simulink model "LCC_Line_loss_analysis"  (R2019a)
settings: Solver=VariableStepAuto  StartTime=0.0  StopTime=10.0  RelTol=1e-3
undefined symbols (not defined in the file or in its folder): D1, Delta
libraries: powerlib x40, powerlib_meascontrol x15

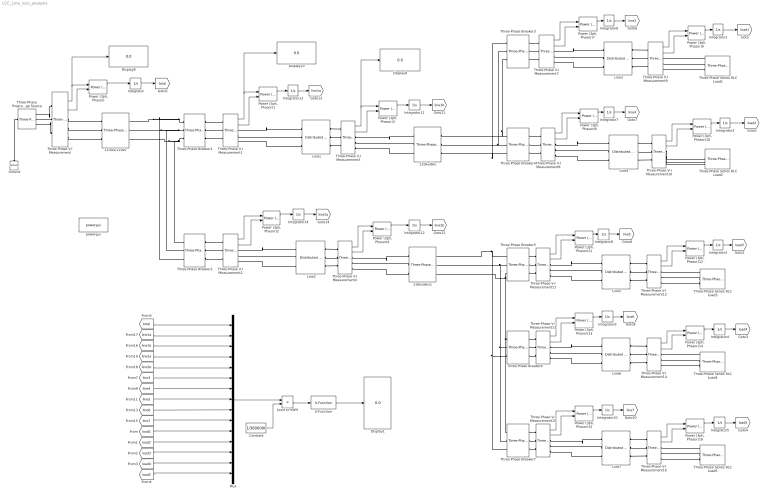
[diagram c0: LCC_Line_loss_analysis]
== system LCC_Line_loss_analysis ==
  " Line1" : powerlib/Elements/Distributed Parameters Line  Phases=3  Frequency=50  Resistance=[0.01273 0.3864]  Inductance="[0.9337e-3  4.1264e-3]"  Capacitance=[12.74e-9 7.751e-9]  Length=50  x1=[2.42627004663306e-09 109999.988635865 109999.988635865;314.159265358979 314.159265358979 314.159265358979;1.80703091597691 0.469420595754554 -1.10137573104034]  x2=[2.86623095915016e-09 110162.552221419 110162.552221419;314.159265358979 314.159265358979 314.159265358979;1.78484613356119 0.469205113607915 -1.10159121318698]  x3=[7.23800122018368e-12 405.078766721455 405.078766721459;314.159265358979 314.159265358979 314.159265358979;0.785734525687869 0.414782441285651 -1.15601388550923]  x4=[7.02816694582336e-12 407.341080813924 407.341080813919;314.159265358979 314.159265358979 314.159265358979;2.98486211281806 0.469482730989694 -1.10131359580521]  x5=0.000282770783497871  V1=[2.426e-09 1.1e+05 1.1e+05;314.2 314.2 314.2;1.807 0.4694 -1.101]  V2=[2.866e-09 1.102e+05 1.102e+05;314.2 314.2 314.2;1.785 0.4692 -1.102]  I1=[7.238e-12 405.1 405.1;314.2 314.2 314.2;0.7857 0.4148 -1.156]  I2=[7.028e-12 407.3 407.3;314.2 314.2 314.2;2.985 0.4695 -1.101]  nHarmo=1  Measurements=None
  " Line2" : powerlib/Elements/Distributed Parameters Line  Phases=3  Frequency=50  Resistance=[0.01273 0.3864]  Inductance="[0.9337e-3  4.1264e-3]"  Capacitance=[12.74e-9 7.751e-9]  Length=50  x1=[2.41365569055271e-09 109999.984096595 109999.984096595;314.159265358979 314.159265358979 314.159265358979;1.810384742463 1.51661814213263 3.08741446892753]  x2=[2.30050693096151e-09 110163.037727826 110163.037727826;314.159265358979 314.159265358979 314.159265358979;1.79045646876788 1.51634195109301 3.08713827788791]  x3=[2.00567277565264e-12 404.628931687138 404.628931687133;314.159265358979 314.159265358979 314.159265358979;2.27601187025823 1.46178814856789 3.03258447536278]  x4=[4.11611761403107e-12 407.795592688783 407.795592688789;314.159265358979 314.159265358979 314.159265358979;1.4069351072644 1.51674944032911 3.08754576712401]  x5=0.000282770783497871  V1=[2.414e-09 1.1e+05 1.1e+05;314.2 314.2 314.2;1.81 1.517 3.087]  V2=[2.301e-09 1.102e+05 1.102e+05;314.2 314.2 314.2;1.79 1.516 3.087]  I1=[2.006e-12 404.6 404.6;314.2 314.2 314.2;2.276 1.462 3.033]  I2=[4.116e-12 407.8 407.8;314.2 314.2 314.2;1.407 1.517 3.088]  nHarmo=1  Measurements=None
  " Line3" : powerlib/Elements/Distributed Parameters Line  Phases=3  Frequency=50  Resistance=[0.01273 0.3864]  Inductance="[0.9337e-3  4.1264e-3]"  Capacitance=[12.74e-9 7.751e-9]  Length=50  x1=[7.59305529381592e-11 6008.18273156121 6008.18273156127;314.159265358979 314.159265358979 314.159265358979;1.15263509813838 0.991548021886359 2.56234434868125]  x2=[6.89253585630512e-11 6010.19477333752 6010.19477333757;314.159265358979 314.159265358979 314.159265358979;1.12473499523216 0.971117638857499 2.54191396565239]  x3=[1.12891283616764e-13 13.8436307559632 13.8436307559631;314.159265358979 314.159265358979 314.159265358979;2.02903845670185 0.918213317671723 2.48900964446667]  x4=[1.94803250183711e-13 30.4994291398562 30.4994291398567;314.159265358979 314.159265358979 314.159265358979;0.741119579924984 0.970570895126736 2.54136722192161]  x5=0.000282770783497871  V1=[7.593e-11 6008 6008;314.2 314.2 314.2;1.153 0.9915 2.562]  V2=[6.893e-11 6010 6010;314.2 314.2 314.2;1.125 0.9711 2.542]  I1=[1.129e-13 13.84 13.84;314.2 314.2 314.2;2.029 0.9182 2.489]  I2=[1.948e-13 30.5 30.5;314.2 314.2 314.2;0.7411 0.9706 2.541]  nHarmo=1  Measurements=None
  " Line4" : powerlib/Elements/Distributed Parameters Line  Phases=3  Frequency=50  Resistance=[0.01273 0.3864]  Inductance="[0.9337e-3  4.1264e-3]"  Capacitance=[12.74e-9 7.751e-9]  Length=100  x1=[7.70769930533368e-11 6008.14875836645 6008.14875836645;314.159265358979 314.159265358979 314.159265358979;0.92815933412839 -0.109826923976571 -1.68062325077146]  x2=[5.61940897329232e-11 6019.23621249713 6019.23621249713;314.159265358979 314.159265358979 314.159265358979;0.4847481944804 -0.167146792126099 -1.73794311892099]  x3=[1.60493033480814e-13 10.5340155159656 10.5340155159655;314.159265358979 314.159265358979 314.159265358979;-3.0013468861881 -0.276666920445539 -1.84746324724043]  x4=[3.57813419959134e-13 33.8325750993465 33.8325750993465;314.159265358979 314.159265358979 314.159265358979;0.332480731404384 -0.166653751439935 -1.73745007823482]  x5=0.000565541566995743  V1=[7.708e-11 6008 6008;314.2 314.2 314.2;0.9282 -0.1098 -1.681]  V2=[5.619e-11 6019 6019;314.2 314.2 314.2;0.4847 -0.1671 -1.738]  I1=[1.605e-13 10.53 10.53;314.2 314.2 314.2;-3.001 -0.2767 -1.847]  I2=[3.578e-13 33.83 33.83;314.2 314.2 314.2;0.3325 -0.1667 -1.737]  nHarmo=1  Measurements=None
  " Line5" : powerlib/Elements/Distributed Parameters Line  Phases=3  Frequency=50  Resistance=[0.01273 0.3864]  Inductance="[0.9337e-3  4.1264e-3]"  Capacitance=[12.74e-9 7.751e-9]  Length=70  x1=[2.06803460954251e-11 6008.01639533854 6008.01639533867;314.159265358979 314.159265358979 314.159265358979;-1.55026791798683 2.01650369223936 -2.69588528814532]  x2=[3.29966131788237e-11 6022.29777272544 6022.29777272558;314.159265358979 314.159265358979 314.159265358979;-2.21431152729356 2.00495247781881 -2.70743650256587]  x3=[2.18092693874683e-13 18.8614244081539 18.8614244081542;314.159265358979 314.159265358979 314.159265358979;2.19365442019187 1.92830769506266 -2.78408128532201]  x4=[2.40433029961128e-13 25.5309379087104 25.5309379087111;314.159265358979 314.159265358979 314.159265358979;-1.27694108346781 2.00560662914093 -2.70678235124375]  x5=0.00039587909689702  V1=[2.068e-11 6008 6008;314.2 314.2 314.2;-1.55 2.017 -2.696]  V2=[3.3e-11 6022 6022;314.2 314.2 314.2;-2.214 2.005 -2.707]  I1=[2.181e-13 18.86 18.86;314.2 314.2 314.2;2.194 1.928 -2.784]  I2=[2.404e-13 25.53 25.53;314.2 314.2 314.2;-1.277 2.006 -2.707]  nHarmo=1  Measurements=None
  " Line6" : powerlib/Elements/Distributed Parameters Line  Phases=3  Frequency=50  Resistance=[0.01273 0.3864]  Inductance="[0.9337e-3  4.1264e-3]"  Capacitance=[12.74e-9 7.751e-9]  Length=75  x1=[1.90824246118878e-11 6007.96613140158 6007.96613140145;314.159265358979 314.159265358979 314.159265358979;-1.26596522315896 0.963888688570127 -0.606907638224758]  x2=[2.76583978250132e-11 6017.39726878102 6017.3972687809;314.159265358979 314.159265358979 314.159265358979;-2.1640200741846 0.933168217076156 -0.637628109718729]  x3=[1.91761145536608e-13 13.8552900858033 13.8552900858031;314.159265358979 314.159265358979 314.159265358979;2.06333552307775 0.850861543484025 -0.719934783310865]  x4=[2.45843562433831e-13 30.5115242564101 30.5115242564094;314.159265358979 314.159265358979 314.159265358979;-1.11015247428008 0.933715077486628 -0.637081249308253]  x5=0.000424156175246807  V1=[1.908e-11 6008 6008;314.2 314.2 314.2;-1.266 0.9639 -0.6069]  V2=[2.766e-11 6017 6017;314.2 314.2 314.2;-2.164 0.9332 -0.6376]  I1=[1.918e-13 13.86 13.86;314.2 314.2 314.2;2.063 0.8509 -0.7199]  I2=[2.458e-13 30.51 30.51;314.2 314.2 314.2;-1.11 0.9337 -0.6371]  nHarmo=1  Measurements=None
  " Line7" : powerlib/Elements/Distributed Parameters Line  Phases=3  Frequency=50  Resistance=[0.01273 0.3864]  Inductance="[0.9337e-3  4.1264e-3]"  Capacitance=[12.74e-9 7.751e-9]  Length=50  x1=[1.81374523428606e-11 6007.88313297421 6007.88313297408;314.159265358979 314.159265358979 314.159265358979;-1.10950345529888 0.990978480375292 -0.579817846419593]  x2=[2.19506880714965e-11 6001.34524535515 6001.34524535502;314.159265358979 314.159265358979 314.159265358979;-1.88953581653548 0.950225697994974 -0.620570628799912]  x3=[1.88636400080801e-13 5.51740302808399 5.51740302808387;314.159265358979 314.159265358979 314.159265358979;2.24025021280838 0.893262455463956 -0.677533871330898]  x4=[2.46025626104762e-13 38.77992905964 38.7799290596392;314.159265358979 314.159265358979 314.159265358979;-1.06174768352794 0.950655064902487 -0.620141261892399]  x5=0.000282770783497871  V1=[1.814e-11 6008 6008;314.2 314.2 314.2;-1.11 0.991 -0.5798]  V2=[2.195e-11 6001 6001;314.2 314.2 314.2;-1.89 0.9502 -0.6206]  I1=[1.886e-13 5.517 5.517;314.2 314.2 314.2;2.24 0.8933 -0.6775]  I2=[2.46e-13 38.78 38.78;314.2 314.2 314.2;-1.062 0.9507 -0.6201]  nHarmo=1  Measurements=None
  110kv/6kv : powerlib/Elements/Three-Phase Transformer (Two Windings)  Winding1Connection=Yg  Winding2Connection=Delta (D1)  CoreType=Three single-phase transformers  SetSaturation=off  Hysteresis=off  DataFile='hysteresis'  SetInitialFlux=off  Measurements=None  UNITS=pu  NominalPower=[ 2e6 , 50 ]  Winding1=[ 110e3 , 0.002 , 0.01]  Winding2=[ 6000 , 0.002 , 0.01]  Rm=500  Lm=500  L0=0.5  Saturation=[ 0,0 ; 0.0024,1.2 ; 1.0,1.52 ]  InitialFluxes=[ 0.8 , -0.8 , 0.7 ]  BreakLoop=off  DiscreteSolver=Trapezoidal iterative  DataType=off  TransfoNumber=1
  110kv/6kv1 : powerlib/Elements/Three-Phase Transformer (Two Windings)  Winding1Connection=Yg  Winding2Connection=Delta (D1)  CoreType=Three single-phase transformers  SetSaturation=off  Hysteresis=off  DataFile='hysteresis'  SetInitialFlux=off  Measurements=None  UNITS=pu  NominalPower=[ 2e6 , 50 ]  Winding1=[ 110e3 , 0.002 , 0.01]  Winding2=[ 6000 , 0.002 , 0.01]  Rm=500  Lm=500  L0=0.5  Saturation=[ 0,0 ; 0.0024,1.2 ; 1.0,1.52 ]  InitialFluxes=[ 0.8 , -0.8 , 0.7 ]  BreakLoop=off  DiscreteSolver=Trapezoidal iterative  DataType=off  TransfoNumber=1
  13.6kv/110kv : powerlib/Elements/Three-Phase Transformer (Two Windings)  Winding1Connection=Y  Winding2Connection=Yg  CoreType=Three single-phase transformers  SetSaturation=off  Hysteresis=off  DataFile='hysteresis'  SetInitialFlux=off  Measurements=None  UNITS=pu  NominalPower=[ 4e6 , 50 ]  Winding1=[ 13600 , 0 , 0]  Winding2=[ 110e3 , 0 , 0]  Rm=inf  Lm=inf  L0=0.5  Saturation=[ 0,0 ; 0.0024,1.2 ; 1.0,1.52 ]  InitialFluxes=[ 0.8 , -0.8 , 0.7 ]  BreakLoop=off  DiscreteSolver=Trapezoidal iterative  DataType=off  TransfoNumber=1
  Constant : Constant  Value=1/3600000
  Display{1,8..10} (4 alike) : Display
  Ground : powerlib/Elements/Ground  LConnTagsString=a
  Integrator{,1..14} (15 alike) : Integrator
  Joule to KWH : Product
  Mux : Mux  Inputs=15
  Power (3ph, Phasor){,1..4,7..16} (15 alike) : powerlib_meascontrol/Measurements/Power (3ph, Phasor)
  S-Function : S-Function  FunctionName=modbusCom2  SFunctionDeploymentMode=off  EnableBusSupport=off
  Three-Phase Programmable Voltage Source : powerlib/Electrical Sources/Three-Phase Programmable Voltage Source  PositiveSequence="[13.6e3  0 50]"  VariationEntity=None  VariationType=Step  VariationTypeAlt=Step  VariationStep=-0.6  VariationRate=10  VariationMagnitude=0.3  VariationFrequency=2  VariationTiming=[20 30]  VariationPhaseA=off  Amplitudes=[1 0.8 1.2 1.0]  TimeValues=[0 0.1 0.15 0.2]  HarmonicGeneration=off  HarmonicA=[3 0.2 -25 0]  HarmonicB=[2 0.15 35 2]  Timing="[0.05  3]"  BusType=swing  Pref=0  Qref=0  Qmin=-inf  Qmax=inf
  Three-Phase Series RLC Load1 : powerlib/Elements/Three-Phase Series RLC Load  LConnTagsString=A|B|C  Configuration=Y (grounded)  NominalVoltage=6000  Vabc=[1e3 1e3 1e3]  Vabcp=[1e3 1e3 1e3]  NominalFrequency=50  UnbalancedPower=off  ActivePower=50000  InductivePower=100  CapacitivePower=0  Pabc=[10e3 9e3 11e3]  QLabc=[100 90 110]  QCabc=[100 90 110]  Pabcp=[10e3 9e3 11e3]  QLabcp=[100 90 110]  QCabcp=[100 90 110]  Measurements=None  LoadType=constant Z
  Three-Phase Series RLC Load2 : powerlib/Elements/Three-Phase Series RLC Load  LConnTagsString=A|B|C  Configuration=Y (grounded)  NominalVoltage=6000  Vabc=[1e3 1e3 1e3]  Vabcp=[1e3 1e3 1e3]  NominalFrequency=50  UnbalancedPower=off  ActivePower=70000  InductivePower=0  CapacitivePower=100  Pabc=[10e3 9e3 11e3]  QLabc=[100 90 110]  QCabc=[100 90 110]  Pabcp=[10e3 9e3 11e3]  QLabcp=[100 90 110]  QCabcp=[100 90 110]  Measurements=None  LoadType=constant PQ
  Three-Phase Series RLC Load3 : powerlib/Elements/Three-Phase Series RLC Load  LConnTagsString=A|B|C  Configuration=Y (grounded)  NominalVoltage=6000  Vabc=[1e3 1e3 1e3]  Vabcp=[1e3 1e3 1e3]  NominalFrequency=50  UnbalancedPower=off  ActivePower=20000  InductivePower=0  CapacitivePower=100  Pabc=[10e3 9e3 11e3]  QLabc=[100 90 110]  QCabc=[100 90 110]  Pabcp=[10e3 9e3 11e3]  QLabcp=[100 90 110]  QCabcp=[100 90 110]  Measurements=None  LoadType=constant Z
  Three-Phase Series RLC Load4 : powerlib/Elements/Three-Phase Series RLC Load  LConnTagsString=A|B|C  Configuration=Y (grounded)  NominalVoltage=6000  Vabc=[1e3 1e3 1e3]  Vabcp=[1e3 1e3 1e3]  NominalFrequency=50  UnbalancedPower=off  ActivePower=50000  InductivePower=0  CapacitivePower=100  Pabc=[10e3 9e3 11e3]  QLabc=[100 90 110]  QCabc=[100 90 110]  Pabcp=[10e3 9e3 11e3]  QLabcp=[100 90 110]  QCabcp=[100 90 110]  Measurements=None  LoadType=constant Z
  Three-Phase Series RLC Load5 : powerlib/Elements/Three-Phase Series RLC Load  LConnTagsString=A|B|C  Configuration=Y (grounded)  NominalVoltage=6000  Vabc=[1e3 1e3 1e3]  Vabcp=[1e3 1e3 1e3]  NominalFrequency=50  UnbalancedPower=off  ActivePower=100000  InductivePower=0  CapacitivePower=100  Pabc=[10e3 9e3 11e3]  QLabc=[100 90 110]  QCabc=[100 90 110]  Pabcp=[10e3 9e3 11e3]  QLabcp=[100 90 110]  QCabcp=[100 90 110]  Measurements=None  LoadType=constant Z
  Three-Phase V-I Measurement{,1..4,7..16} (15 alike) : powerlib/Measurements/Three-Phase V-I Measurement  VoltageMeasurement=phase-to-ground  SetLabelV=off  LabelV=Vabc  Vpu=off  VpuLL=off  CurrentMeasurement=yes  SetLabelI=off  LabelI=Iabc  Ipu=off  Pbase=100e6  Vbase=500e3  OutputType=Complex  PhasorSimulation=off  PSBequivalent=0
  Three-Phase Breaker{1..7} (7 alike) : powerlib/Elements/Three-Phase Breaker  InitialState=closed  SwitchA=on  SwitchB=on  SwitchC=on  SwitchTimes=10  External=off  BreakerResistance=0.01  SnubberResistance=1e6  SnubberCapacitance=inf  Measurements=None
  powergui : powerlib/powergui  Priority=1  SimulationMode=Continuous  SampleTime=50e-6  frequency=60  Iterations=50  frequencyindice=50  Pbase=100e6  ErrMax=1e-4  UnitsV=kV  UnitsW=MW  buscounter=0  FunctionMessages=off  echomessages=off  EnableUseOfTLC=off  CurrentSourceSwitches=off  DisableSnubberDevices=off  DisableRonSwitches=off  DisableVfSwitches=off  DisplayEquations=off  AutomaticDiscreteSolvers=off  SolverType=Tustin/Backward Euler (TBE)  Interpol=off  ExternalGateDelay=off  methode=off  Ts=100  x0status=blocks  SPID=on  SwTol=0  HookPort=off  NonlinearTolerance=1e-4  nMaxIteration=100  ContinueOnMaxIteration=off  RestoreLinks=warning  ResistiveCurrentMeasurement=off  Frange=[0:2:500]  Ylog=off  Xlog=on  ShowGrid=off  save=off  variable=ZData  structure=0  ZoomFFT=off  StartTime=0.0  cycles=1  DisplayStyle=1  fundamental=60  FreqAxis=off  MaxFrequency=1000  frequencyindicesteady=1  RmsSteady=1  display=off
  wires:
  [load4] -> Mux/14
  S-Function/1 -> Display1/1
  [line2a] -> Mux/4
  [line5] -> Mux/8
  [line1b] -> Mux/3
  [line1a] -> Mux/2
  [line4] -> Mux/7
  [load3] -> Mux/13
  [load2] -> Mux/12
  [line7] -> Mux/10
  [line2b] -> Mux/5
  [total] -> Mux/1
  Constant/1 -> Joule to KWH/2
  Joule to KWH/1 -> S-Function/1
  [load1] -> Mux/11
  [line6] -> Mux/9
  [load5] -> Mux/15
  [line3] -> Mux/6
  Mux/1 -> Joule to KWH/1
  Three-Phase V-I Measurement12/2 -> "Power (3ph, Phasor)12"/2
  "Power (3ph, Phasor)13"/1 -> Integrator9/1
  Three-Phase V-I Measurement1/2 -> "Power (3ph, Phasor)1"/2
  Integrator10/1 -> [line7]
  "Power (3ph, Phasor)7"/1 -> Integrator6/1
  Three-Phase V-I Measurement11/1 -> "Power (3ph, Phasor)11"/1
  Three-Phase V-I Measurement15/1 -> "Power (3ph, Phasor)15"/1
  "Power (3ph, Phasor)15"/1 -> Integrator10/1
  Integrator9/1 -> [line6]
  Three-Phase V-I Measurement16/1 -> "Power (3ph, Phasor)16"/1
  Integrator/1 -> [total]
  Three-Phase V-I Measurement15/2 -> "Power (3ph, Phasor)15"/2
  Three-Phase V-I Measurement14/2 -> "Power (3ph, Phasor)14"/2
  Three-Phase V-I Measurement14/1 -> "Power (3ph, Phasor)14"/1
  Integrator14/1 -> [line2a]
  Three-Phase V-I Measurement1/1 -> Display10/1, "Power (3ph, Phasor)1"/1
  Three-Phase V-I Measurement10/1 -> "Power (3ph, Phasor)10"/1
  Three-Phase V-I Measurement10/2 -> "Power (3ph, Phasor)10"/2
  Three-Phase V-I Measurement12/1 -> "Power (3ph, Phasor)12"/1
  Integrator6/1 -> [line3]
  Three-Phase V-I Measurement13/1 -> "Power (3ph, Phasor)13"/1
  "Power (3ph, Phasor)12"/1 -> Integrator3/1
  "Power (3ph, Phasor)2"/1 -> Integrator14/1
  "Power (3ph, Phasor)11"/1 -> Integrator8/1
  Three-Phase V-I Measurement13/2 -> "Power (3ph, Phasor)13"/2
  "Power (3ph, Phasor)9"/1 -> Integrator1/1
  Three-Phase V-I Measurement8/1 -> "Power (3ph, Phasor)8"/1
  Three-Phase V-I Measurement2/1 -> "Power (3ph, Phasor)2"/1
  "Power (3ph, Phasor)10"/1 -> Integrator2/1
  "Power (3ph, Phasor)8"/1 -> Integrator7/1
  Three-Phase V-I Measurement3/2 -> "Power (3ph, Phasor)3"/2
  Integrator8/1 -> [line5]
  Three-Phase V-I Measurement16/2 -> "Power (3ph, Phasor)16"/2
  Three-Phase V-I Measurement9/1 -> "Power (3ph, Phasor)9"/1
  Integrator7/1 -> [line4]
  Three-Phase V-I Measurement9/2 -> "Power (3ph, Phasor)9"/2
  "Power (3ph, Phasor)4"/1 -> Integrator12/1
  Three-Phase V-I Measurement8/2 -> "Power (3ph, Phasor)8"/2
  "Power (3ph, Phasor)1"/1 -> Integrator13/1
  Three-Phase V-I Measurement2/2 -> "Power (3ph, Phasor)2"/2
  Three-Phase V-I Measurement/1 -> Display8/1, "Power (3ph, Phasor)"/1
  Three-Phase V-I Measurement7/1 -> "Power (3ph, Phasor)7"/1
  Integrator12/1 -> [line2b]
  Three-Phase V-I Measurement11/2 -> "Power (3ph, Phasor)11"/2
  Integrator13/1 -> [line1a]
  Integrator5/1 -> [load5]
  Three-Phase V-I Measurement/2 -> "Power (3ph, Phasor)"/2
  Integrator4/1 -> [load4]
  "Power (3ph, Phasor)3"/1 -> Integrator11/1
  Integrator1/1 -> [load1]
  Integrator11/1 -> [line1b]
  Three-Phase V-I Measurement4/1 -> "Power (3ph, Phasor)4"/1
  Integrator2/1 -> [load2]
  "Power (3ph, Phasor)16"/1 -> Integrator5/1
  "Power (3ph, Phasor)"/1 -> Integrator/1
  Three-Phase V-I Measurement7/2 -> "Power (3ph, Phasor)7"/2
  Three-Phase V-I Measurement3/1 -> Display9/1, "Power (3ph, Phasor)3"/1
  Integrator3/1 -> [load3]
  "Power (3ph, Phasor)14"/1 -> Integrator4/1
  Three-Phase V-I Measurement4/2 -> "Power (3ph, Phasor)4"/2
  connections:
  Three-Phase Breaker6/LConn1 -- 110kv/6kv1/RConn3 -- Three-Phase Breaker5/LConn3 -- Three-Phase Breaker7/LConn1
  Three-Phase Breaker1/LConn3 -- Three-Phase Breaker2/LConn1 -- 13.6kv/110kv/RConn3
  Three-Phase Breaker1/LConn2 -- Three-Phase Breaker2/LConn2 -- 13.6kv/110kv/RConn2
  Three-Phase Breaker3/LConn2 -- 110kv/6kv/RConn2 -- Three-Phase Breaker4/LConn2
  Three-Phase Breaker7/LConn2 -- 110kv/6kv1/RConn2 -- Three-Phase Breaker5/LConn2 -- Three-Phase Breaker6/LConn2
  Three-Phase Breaker3/LConn1 -- 110kv/6kv/RConn3 -- Three-Phase Breaker4/LConn3
  Three-Phase Breaker6/LConn3 -- 110kv/6kv1/RConn1 -- Three-Phase Breaker5/LConn1 -- Three-Phase Breaker7/LConn3
  Three-Phase Breaker3/LConn3 -- 110kv/6kv/RConn1 -- Three-Phase Breaker4/LConn1
  Three-Phase Breaker1/LConn1 -- Three-Phase Breaker2/LConn3 -- 13.6kv/110kv/RConn1
  Three-Phase Series RLC Load5/LConn1 -- Three-Phase V-I Measurement16/RConn1
  " Line7"/LConn1 -- Three-Phase V-I Measurement15/RConn1
  " Line3"/RConn3 -- Three-Phase V-I Measurement9/LConn3
  Three-Phase Series RLC Load4/LConn3 -- Three-Phase V-I Measurement14/RConn3
  Three-Phase V-I Measurement16/LConn2 -- " Line7"/RConn2
  Three-Phase V-I Measurement13/RConn1 -- " Line6"/LConn1
  Three-Phase V-I Measurement7/RConn1 -- " Line3"/LConn1
  110kv/6kv/LConn2 -- Three-Phase V-I Measurement3/RConn2
  Three-Phase V-I Measurement15/LConn1 -- Three-Phase Breaker7/RConn1
  Three-Phase V-I Measurement1/RConn1 -- " Line1"/LConn1
  Three-Phase V-I Measurement16/LConn3 -- " Line7"/RConn3
  Three-Phase V-I Measurement11/RConn3 -- " Line5"/LConn3
  Three-Phase V-I Measurement16/LConn1 -- " Line7"/RConn1
  Three-Phase V-I Measurement3/LConn2 -- " Line1"/RConn2
  Three-Phase V-I Measurement11/RConn1 -- " Line5"/LConn1
  Three-Phase V-I Measurement8/LConn3 -- Three-Phase Breaker4/RConn3
  Three-Phase V-I Measurement7/RConn3 -- " Line3"/LConn3
  Three-Phase V-I Measurement11/LConn1 -- Three-Phase Breaker5/RConn1
  Three-Phase Breaker1/RConn1 -- Three-Phase V-I Measurement1/LConn1
  Three-Phase V-I Measurement9/LConn1 -- " Line3"/RConn1
  Three-Phase V-I Measurement10/LConn2 -- " Line4"/RConn2
  Three-Phase V-I Measurement2/LConn3 -- Three-Phase Breaker2/RConn3
  Three-Phase Series RLC Load4/LConn1 -- Three-Phase V-I Measurement14/RConn1
  Three-Phase V-I Measurement10/LConn1 -- " Line4"/RConn1
  Three-Phase V-I Measurement15/LConn3 -- Three-Phase Breaker7/RConn3
  Three-Phase V-I Measurement15/LConn2 -- Three-Phase Breaker7/RConn2
  Three-Phase V-I Measurement13/LConn2 -- Three-Phase Breaker6/RConn2
  Three-Phase V-I Measurement11/LConn3 -- Three-Phase Breaker5/RConn3
  Three-Phase V-I Measurement14/LConn3 -- " Line6"/RConn3
  Three-Phase Series RLC Load1/LConn2 -- Three-Phase V-I Measurement9/RConn2
  " Line6"/LConn2 -- Three-Phase V-I Measurement13/RConn2
  Three-Phase V-I Measurement1/RConn3 -- " Line1"/LConn3
  Three-Phase V-I Measurement4/LConn1 -- " Line2"/RConn1
  Three-Phase V-I Measurement14/LConn2 -- " Line6"/RConn2
  Three-Phase Breaker1/RConn3 -- Three-Phase V-I Measurement1/LConn3
  " Line7"/LConn2 -- Three-Phase V-I Measurement15/RConn2
  Three-Phase Series RLC Load3/LConn2 -- Three-Phase V-I Measurement12/RConn2
  " Line3"/RConn2 -- Three-Phase V-I Measurement9/LConn2
  Three-Phase Series RLC Load1/LConn1 -- Three-Phase V-I Measurement9/RConn1
  Three-Phase V-I Measurement8/LConn1 -- Three-Phase Breaker4/RConn1
  Three-Phase V-I Measurement11/LConn2 -- Three-Phase Breaker5/RConn2
  Ground/LConn1 -- Three-Phase Programmable Voltage Source/LConn1
  Three-Phase V-I Measurement13/RConn3 -- " Line6"/LConn3
  Three-Phase V-I Measurement7/LConn2 -- Three-Phase Breaker3/RConn2
  Three-Phase V-I Measurement14/LConn1 -- " Line6"/RConn1
  Three-Phase V-I Measurement13/LConn3 -- Three-Phase Breaker6/RConn3
  Three-Phase V-I Measurement7/LConn1 -- Three-Phase Breaker3/RConn1
  Three-Phase V-I Measurement8/RConn3 -- " Line4"/LConn3
  Three-Phase V-I Measurement3/LConn1 -- " Line1"/RConn1
  Three-Phase V-I Measurement10/RConn3 -- Three-Phase Series RLC Load2/LConn3
  Three-Phase Series RLC Load3/LConn1 -- Three-Phase V-I Measurement12/RConn1
  Three-Phase V-I Measurement/LConn1 -- Three-Phase Programmable Voltage Source/RConn1
  Three-Phase V-I Measurement10/LConn3 -- " Line4"/RConn3
  " Line3"/LConn2 -- Three-Phase V-I Measurement7/RConn2
  Three-Phase V-I Measurement10/RConn1 -- Three-Phase Series RLC Load2/LConn1
  " Line4"/LConn2 -- Three-Phase V-I Measurement8/RConn2
  Three-Phase V-I Measurement8/RConn1 -- " Line4"/LConn1
  Three-Phase Breaker1/RConn2 -- Three-Phase V-I Measurement1/LConn2
  Three-Phase Series RLC Load1/LConn3 -- Three-Phase V-I Measurement9/RConn3
  Three-Phase V-I Measurement/RConn2 -- 13.6kv/110kv/LConn2
  Three-Phase V-I Measurement4/LConn2 -- " Line2"/RConn2
  Three-Phase Programmable Voltage Source/RConn2 -- Three-Phase V-I Measurement/LConn2
  " Line5"/LConn2 -- Three-Phase V-I Measurement11/RConn2
  Three-Phase V-I Measurement2/LConn1 -- Three-Phase Breaker2/RConn1
  Three-Phase Series RLC Load4/LConn2 -- Three-Phase V-I Measurement14/RConn2
  Three-Phase V-I Measurement13/LConn1 -- Three-Phase Breaker6/RConn1
  Three-Phase V-I Measurement/RConn3 -- 13.6kv/110kv/LConn3
  Three-Phase Series RLC Load5/LConn2 -- Three-Phase V-I Measurement16/RConn2
  Three-Phase V-I Measurement/RConn1 -- 13.6kv/110kv/LConn1
  Three-Phase V-I Measurement12/LConn3 -- " Line5"/RConn3
  Three-Phase V-I Measurement/LConn3 -- Three-Phase Programmable Voltage Source/RConn3
  Three-Phase V-I Measurement3/LConn3 -- " Line1"/RConn3
  Three-Phase V-I Measurement8/LConn2 -- Three-Phase Breaker4/RConn2
  Three-Phase V-I Measurement7/LConn3 -- Three-Phase Breaker3/RConn3
  110kv/6kv1/LConn1 -- Three-Phase V-I Measurement4/RConn1
  110kv/6kv1/LConn3 -- Three-Phase V-I Measurement4/RConn3
  110kv/6kv1/LConn2 -- Three-Phase V-I Measurement4/RConn2
  Three-Phase V-I Measurement2/LConn2 -- Three-Phase Breaker2/RConn2
  Three-Phase V-I Measurement15/RConn3 -- " Line7"/LConn3
  110kv/6kv/LConn1 -- Three-Phase V-I Measurement3/RConn1
  110kv/6kv/LConn3 -- Three-Phase V-I Measurement3/RConn3
  Three-Phase Series RLC Load5/LConn3 -- Three-Phase V-I Measurement16/RConn3
  Three-Phase V-I Measurement12/LConn2 -- " Line5"/RConn2
  Three-Phase V-I Measurement2/RConn1 -- " Line2"/LConn1
  " Line2"/RConn3 -- Three-Phase V-I Measurement4/LConn3
  Three-Phase V-I Measurement1/RConn2 -- " Line1"/LConn2
  Three-Phase V-I Measurement12/LConn1 -- " Line5"/RConn1
  Three-Phase Series RLC Load3/LConn3 -- Three-Phase V-I Measurement12/RConn3
  " Line2"/LConn2 -- Three-Phase V-I Measurement2/RConn2
  Three-Phase V-I Measurement2/RConn3 -- " Line2"/LConn3
  Three-Phase V-I Measurement10/RConn2 -- Three-Phase Series RLC Load2/LConn2
